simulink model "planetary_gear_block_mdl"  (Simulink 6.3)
settings: Solver=ode45  StartTime=0.0  StopTime=3  RelTol=1e-3
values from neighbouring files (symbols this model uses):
  b_c = kb*J_c    (= 92.8974810391)    [architetture_epicicloidale_statico.m]    (also in architetture_HEV_startstop_1.m = 9.28974810391; architetture_HEV_startstop_2.m = 9.28974810391; architetture_epicicloidale.m = 4.94590955184; architetture_epicicloidale_cont.m = 4.94590955184)
  b_p = kb*J_p    (= 8.12277148259)    [architetture_epicicloidale_statico.m]    (also in architetture_HEV_startstop_1.m = 0.812277148259; architetture_HEV_startstop_2.m = 0.812277148259; CVT_New.m = 0.00430287434624; CVT_New_th.m = 0.00430287434624)
  b_r = kb*J_r    (= 218.026030555)    [architetture_epicicloidale_statico.m]    (also in architetture_HEV_startstop_1.m = 21.8026030555; architetture_HEV_startstop_2.m = 21.8026030555; CVT_New.m = 0.218026030555; CVT_New_th.m = 0.218026030555)
  b_s = kb*J_s    (= 4.94590955184)    [architetture_epicicloidale_statico.m]    (also in architetture_HEV_startstop_1.m = 0.494590955184; architetture_HEV_startstop_2.m = 0.494590955184; CVT_New.m = 0.0104441563023; CVT_New_th.m = 0.0104441563023)
  d_cr = d0    (= 1000)    [architetture_HEV_startstop_1.m]    (also in architetture_HEV_startstop_2.m; architetture_epicicloidale_HEV.m = 10; architetture_HEV_controllo.m; architetture_HEV_startstop.m = 90)
  d_sc = d0    (= 1000)    [architetture_HEV_startstop_1.m]    (also in architetture_HEV_startstop_2.m; architetture_epicicloidale_HEV.m = 10; architetture_HEV_controllo.m; architetture_HEV_startstop.m = 90)
  J_c = Nr_sat*(r_s+r_p)^2*rho_acc*pi*(hs*r_p^2 + hc*r_p^2)    (= 0.928974810391)    [architetture_epicicloidale_statico.m]    (also in architetture_HEV_startstop_1.m; architetture_HEV_startstop_2.m; architetture_epicicloidale.m = 0.0494590955184; architetture_epicicloidale_cont.m = 0.0494590955184)
  J_p = Nr_sat*0.5*pi*rho_acc*(hs*r_p^4 + hc*r_p^4)    (= 0.0812277148259)    [architetture_epicicloidale_statico.m]    (also in architetture_HEV_startstop_1.m; architetture_HEV_startstop_2.m; CVT_New.m = 4.30287434624e-05; CVT_New_th.m = 4.30287434624e-05)
  J_r = 0.5*pi*rho_acc*(hr*r_r^4 + h_ring*(r_re^4-r_r^4))    (= 2.18026030555)    [architetture_epicicloidale_statico.m]    (also in architetture_HEV_startstop_1.m; architetture_HEV_startstop_2.m; CVT_New.m = 0.00218026030555; CVT_New_th.m = 0.00218026030555)
  J_s = 1.3*0.5*pi*rho_acc*hc*r_s^4    (= 0.0494590955184)    [architetture_epicicloidale_statico.m]    (also in architetture_HEV_startstop_1.m; architetture_HEV_startstop_2.m; CVT_New.m = 0.000104441563023; CVT_New_th.m = 0.000104441563023)
  K_cr = K0    (= 10000000)    [architetture_HEV_startstop_1.m]    (also in architetture_HEV_startstop_2.m; architetture_epicicloidale_HEV.m = 10000; architetture_HEV_controllo.m = 100000; architetture_HEV_startstop.m)
  K_sc = K0    (= 10000000)    [architetture_HEV_startstop_1.m]    (also in architetture_HEV_startstop_2.m; architetture_epicicloidale_HEV.m = 10000; architetture_HEV_controllo.m = 100000; architetture_HEV_startstop.m)
  Nr_sat = 4    [architetture_epicicloidale_statico.m]    (also in architetture_HEV_startstop_1.m; architetture_HEV_startstop_2.m; architetture_epicicloidale.m; architetture_epicicloidale_cont.m)
  r_p = xds*Np/(2*pi)    (= 0.0732112738223)    [architetture_epicicloidale_statico.m]    (also in architetture_HEV_startstop_1.m; architetture_HEV_startstop_2.m; CVT_New.m = 0.105042262441; CVT_New_th.m = 0.105042262441)
  r_r = xds*Nr/(2*pi)    (= 0.248281711223)    [architetture_epicicloidale_statico.m]    (also in architetture_HEV_startstop_1.m; architetture_HEV_startstop_2.m; architetture_epicicloidale_HEV.m; architetture_HEV_controllo.m)
  r_s = r_r-2*r_p    (= 0.101859163579)    [architetture_epicicloidale_statico.m]    (also in architetture_HEV_startstop_1.m; architetture_HEV_startstop_2.m; architetture_epicicloidale.m = 0.0732112738223; architetture_epicicloidale_cont.m = 0.0732112738223)
  Tau_c = 0*N*metri    (= 0)    [architetture_epicicloidale_statico.m]    (also in architetture_epicicloidale.m; architetture_epicicloidale_cont.m; architetture_epicicloidale_prova.m; epicicloidale.m)
  Tau_r = 0*N*metri    (= 0)    [architetture_epicicloidale_statico.m]    (also in architetture_epicicloidale.m; architetture_epicicloidale_cont.m; architetture_epicicloidale_prova.m; epicicloidale.m)
  Tau_s = 5*N*metri    (= 5)    [epicicloidale_confronto_statico_elastico.m]    (also in epicicloidale_statico.m = 0)
  Tc = 0.05*ms    (= 5e-05)    [architetture_epicicloidale_statico.m]    (also in architetture_HEV_startstop_1.m; architetture_HEV_startstop_2.m; CVT_New.m; CVT_New_th.m)
  Wc_0 = -0*0.2*rad/secondo    (= 0)    [architetture_epicicloidale_statico.m]    (also in architetture_epicicloidale.m; architetture_epicicloidale_cont.m; architetture_epicicloidale_HEV.m; architetture_epicicloidale_prova.m)
  Wr_0 = WW_0(5),    [CVT_New.m]    (also in CVT_New_th.m; architetture_epicicloidale.m = Sys1.C(3,:)*[Wc_0; Wsc_0]; Confronto_CVT_EMR.m = 0; epicicloidale.m = Sys1.C(3,:)*[Wc_0; Wsc_0])
  Ws_0 = 0*0.1*rad/secondo    (= 0)    [architetture_epicicloidale_statico.m]    (also in epicicloidale_confronto_statico_elastico.m = 0.1; epicicloidale_statico.m = 0.1)
undefined symbols (not defined in the file or in its folder): Tau3, W1, W2

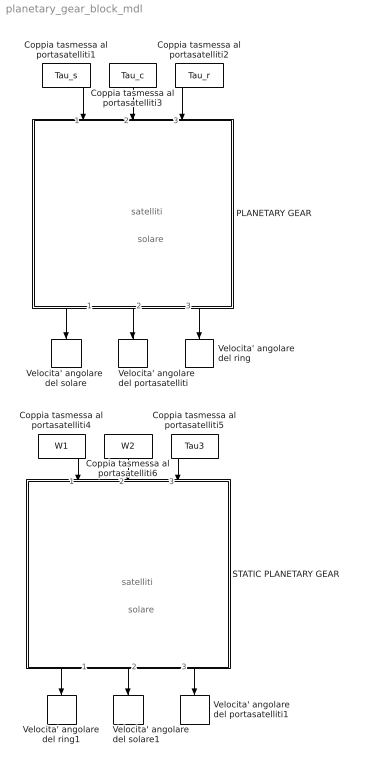
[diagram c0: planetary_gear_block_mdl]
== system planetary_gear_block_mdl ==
  note: solare
  note: satelliti
  note: solare
  note: satelliti
  Coppia tasmessa al portasatelliti1 : Constant  Orientation=down  Value=Tau_s
  Coppia tasmessa al portasatelliti2 : Constant  Orientation=down  Value=Tau_r
  Coppia tasmessa al portasatelliti3 : Constant  Orientation=down  Value=Tau_c
  Coppia tasmessa al portasatelliti4 : Constant  Orientation=down  Value=W1
  Coppia tasmessa al portasatelliti5 : Constant  Orientation=down  Value=Tau3
  Coppia tasmessa al portasatelliti6 : Constant  Orientation=down  Value=W2
  PLANETARY GEAR : Subsystem  Orientation=down  mask(POG Gruppo epicicloidale){Par_solare=[J_s, b_s, r_s], Par_satelliti=[J_p, J_c, b_p, b_c, r_p, Nr_sat], Par_ring=[J_r, b_r, r_r], Tipo_di_Modello=Modello ridotto Ws-Wc, Cond_in_Ws_Wc=[Ws_0,  Wc_0], Cond_in_Wc_Wr=[Wc_0,  Wr_0], Cond_in_Ws_Wr=[Ws_0,  Wr_0], Solare_Satelliti=[K_sc, d_sc], Satelliti_Ring=[K_cr, d_cr], Cond_in=[Ws_0, Wc_0, Wr_0]}
      mask prompts: Par_solare "Parametri Solare: [J_s, b_s, r_s]-->[kg*m^2,N*m*s/rad,m]"; Par_satelliti "Parametri Satelliti: [J_p, J_c, b_p, b_c, r_p, Nr_sat]-->[kg*m^2,N*m*s/rad,m]"; Par_ring "Parametri Ring: [J_r, b_r, r_r]-->[kg*m^2,N*m*s/rad,m,m]"; Tipo_di_Modello "Tipo di modello"; Cond_in_Ws_Wc "Condizioni iniziali: [Ws_0,  Wc_0]-->[rad/s]"; Cond_in_Wc_Wr "Condizioni iniziali: [Wc_0,  Wr_0]-->[rad/s]"; Cond_in_Ws_Wr "Condizioni iniziali: [Ws_0,  Wr_0]-->[rad/s]"; Solare_Satelliti "Solare-Satelliti: [K_sc, d_sc]-->[N/m,N*m*s/rad]"; Satelliti_Ring "Satelliti-Ring: [K_cr, d_cr]-->[N/m,N*m*s/rad]"; Cond_in "Condizioni iniziali: [Ws_0,  Wc_0, Wr_0]-->[rad/s]"
      mask help: Gruppo epicicloidale: [J_s, J_p, J_c, J_r]= Inerzie di: solare, satelliti, porta-satelliti, ring; [b_s, b_p, b_c, b_r]= Attriti di: solare, satelliti, porta-satelliti, ring; [r_s, r_p, r_r]= Raggi di: solare, satelliti, ring; [Nr_sat]= Numero Satelliti; [K_sc, K_cr]= Elasticita' tra solare-satelliti e tra satelliti-ring; [d_sc, d_cr]= Elementi della matrice D; [Ws_0, Wc_0, Wr_0]=Velocita' iniziali di solare, porta-satelliti, ring;
      mask init:
      | J_s=double(Par_solare(1));          
      | b_s=double(Par_solare(2));            
      | r_s=double(Par_solare(3));           
      | %
      | J_p=double(Par_satelliti(1));            
      | J_c=double(Par_satelliti(2));            
      | b_p=double(Par_satelliti(3));            
      | b_c=double(Par_satelliti(4));            
      | r_p=double(Par_satelliti(5));            
      | Nr_sat=double(Par_satelliti(6));           
      | %
      | J_r=double(Par_ring(1));             
      | b_r=double(Par_ring(2));            
      | r_r=double(Par_ring(3));                  
      | %
      | %%%%%%%%%%%%%%%%%%%%%%%%%%%%%%%%%%%%%%%%%%%%%%%%%%%%%%%%%%%%%%%%%%%%%%%%%%%
      | %   Modello esteso e modelli ridotti
      | %%%%%%%%%%%%%%%%%%%%%%%%%%%%%%%%%%%%%%%%%%%%%%%%%%%%%%%%%%%%%%%%%%%%%%%%%%%
      | if Tipo_di_Modello=='Modello esteso       '
      |     %
      |     K_sc=double(Solare_Satelliti(1));
      |     d_sc=double(Solare_Satelliti(2));
      |     if(K_sc==0)
      |         K_sc=inf;
      |     end
      |     %
      |     K_cr=double(Satelliti_Ring(1));
      |     d_cr=double(Satelliti_Ring(2));
      |     if(K_cr==0)
      |         K_cr=inf;
      |     end
      |     %
      |     %
      |     L=[ J_s,    0,      0,      0,      0,      0;
      |         0, 1/K_sc,      0,      0,      0,      0;
      |         0,      0,    J_p,      0,      0,      0;
      |         0,      0,      0,    J_c,      0,      0;
      |         0,      0,      0,      0, 1/K_cr,      0;
      |         0,      0,      0,      0,      0,    J_r];
      |     %
      |     A=- [-b_s-r_s^2*d_sc,                       -r_s,              -r_s*d_sc*r_p,                 r_s^2*d_sc,                          0,                          0;
      |                         r_s,                          0,                        r_p,                       -r_s,                          0,                          0;
      |               -r_s*d_sc*r_p,                       -r_p, -b_p-d_sc*r_p^2-d_cr*r_p^2,  r_s*d_sc*r_p-d_cr*r_p*r_r,                       -r_p,               d_cr*r_p*r_r;
      |                  r_s^2*d_sc,                        r_s,  r_s*d_sc*r_p-d_cr*r_p*r_r, -b_c-r_s^2*d_sc-d_cr*r_r^2,                       -r_r,                 d_cr*r_r^2;
      |                           0,                          0,                        r_p,                        r_r,                          0,                       -r_r;
      |                           0,                          0,               d_cr*r_p*r_r,                 d_cr*r_r^2,                        r_r,            -b_r-d_cr*r_r^2];
      | %                         
      |     B=[ 1, 0, 0;
      |         0, 0, 0;
      |         0, 0, 0;
      |         0, 1, 0;
      |         0, 0, 0;
      |         0, 0, 1];
      |     %
      |     C=[ 1, 0, 0, 0, 0, 0;
      |         0, 0, 0, 1, 0, 0;
      |         0, 0, 0, 0, 0, 1];
      |     %
      |     Ws_0=double(Cond_in(1));
      |     Wc_0=double(Cond_in(2));
      |     Wr_0=double(Cond_in(3));
      |     Wp_0=r_s*(Wc_0-Ws_0)/r_p;
      |     Wpc_0=[Wp_0 Wc_0];
      |     %
      |     We_0=[Ws_0 0 Wpc_0 0 Wr_0 ];
      |     %
      | elseif Tipo_di_Modello=='Modello ridotto Ws-Wc'
      |     L = [(J_s*r_p^2*r_r^2+r_s^2*J_p*r_r^2+r_s^2*J_r*r_p^2)/r_p^2/r_r^2,                                      -r_s*(r_s*J_p*r_r^2+J_r*r_p^2*r_s+J_r*r_p^2*r_r)/r_p^2/r_r^2;
      |            -r_s*(r_s*J_p*r_r^2+J_r*r_p^2*r_s+J_r*r_p^2*r_r)/r_p^2/r_r^2, (J_c*r_p^2*r_r^2+r_s^2*J_p*r_r^2+r_s^2*J_r*r_p^2+2*J_r*r_p^2*r_s*r_r+J_r*r_p^2*r_r^2)/r_p^2/r_r^2];
      |     %
      |     A=-[ -(b_s*r_p^2*r_r^2+r_s^2*b_p*r_r^2+r_s^2*b_r*r_p^2)/r_p^2/r_r^2,                                        r_s*(r_s*b_p*r_r^2+b_r*r_p^2*r_s+b_r*r_p^2*r_r)/r_p^2/r_r^2;
      |         r_s*(r_s*b_p*r_r^2+b_r*r_p^2*r_s+b_r*r_p^2*r_r)/r_p^2/r_r^2, -(b_c*r_p^2*r_r^2+r_s^2*b_p*r_r^2+r_s^2*b_r*r_p^2+2*b_r*r_p^2*r_s*r_r+b_r*r_p^2*r_r^2)/r_p^2/r_r^2];
      |     %
      |     B= [  1,             0,    -1/r_r*r_s;
      |            0,             1, (r_s+r_r)/r_r];
      |     %
      |     C= [            1,               0;
      |                     0,               1;
      |            -1/r_r*r_s, (r_s+r_r)/r_r];
      |     %
      |     Ws_0=double(Cond_in_Ws_Wc(1));
      |     Wc_0=double(Cond_in_Ws_Wc(2));
      |     We_0=[Ws_0 Wc_0];
      |     %
      | elseif Tipo_di_Modello=='Modello ridotto Wc-Wr'
      |     L= [ (J_c*r_s^2*r_p^2+J_s*r_p^2*r_s^2+2*J_s*r_p^2*r_s*r_r+J_s*r_p^2*r_r^2+r_r^2*J_p*r_s^2)/r_s^2/r_p^2,                                      -r_r*(J_s*r_p^2*r_s+J_s*r_p^2*r_r+r_r*J_p*r_s^2)/r_s^2/r_p^2;
      |           -r_r*(J_s*r_p^2*r_s+J_s*r_p^2*r_r+r_r*J_p*r_s^2)/r_s^2/r_p^2,                                     (J_r*r_s^2*r_p^2+J_s*r_p^2*r_r^2+r_r^2*J_p*r_s^2)/r_s^2/r_p^2];
      | 
      |     A=-[  -(b_c*r_s^2*r_p^2+b_s*r_p^2*r_s^2+2*b_s*r_p^2*r_s*r_r+b_s*r_p^2*r_r^2+r_r^2*b_p*r_s^2)/r_s^2/r_p^2,                                        r_r*(b_s*r_p^2*r_s+b_s*r_p^2*r_r+r_r*b_p*r_s^2)/r_s^2/r_p^2;
      |          r_r*(b_s*r_p^2*r_s+b_s*r_p^2*r_r+r_r*b_p*r_s^2)/r_s^2/r_p^2,                                     -(b_r*r_s^2*r_p^2+b_s*r_p^2*r_r^2+r_r^2*b_p*r_s^2)/r_s^2/r_p^2];
      | 
      |     B= [ (r_s+r_r)/r_s,    1,   0;
      |             -1/r_s*r_r,    0,   1];
      | 
      |     C= [ (r_s+r_r)/r_s,    -1/r_s*r_r;
      |                       1,            0;
      |                       0,            1];
      |     %
      |     Wc_0=double(Cond_in_Wc_Wr(1));
      |     Wr_0=double(Cond_in_Wc_Wr(2));
      |     We_0=[Wc_0 Wr_0];
      |     %
      | elseif Tipo_di_Modello=='Modello ridotto Ws-Wr'
      |     L= [ (J_c*r_s^2*r_p^2+J_s*r_p^2*r_s^2+2*J_s*r_p^2*r_s*r_r+J_s*r_p^2*r_r^2+r_r^2*J_p*r_s^2)/r_p^2/(r_s+r_r)^2,                                                      -r_s*r_r*(r_r*J_p*r_s-J_c*r_p^2)/r_p^2/(r_s+r_r)^2;
      |           -r_s*r_r*(r_r*J_p*r_s-J_c*r_p^2)/r_p^2/(r_s+r_r)^2, (J_r*r_s^2*r_p^2+2*J_r*r_p^2*r_s*r_r+J_r*r_p^2*r_r^2+r_r^2*J_p*r_s^2+r_r^2*J_c*r_p^2)/r_p^2/(r_s+r_r)^2];
      | 
      |     A=-[-(b_c*r_s^2*r_p^2+b_s*r_p^2*r_s^2+2*b_s*r_p^2*r_s*r_r+b_s*r_p^2*r_r^2+r_r^2*b_p*r_s^2)/r_p^2/(r_s+r_r)^2,                                                      -r_s*r_r*(-r_s*r_r*b_p+r_p^2*b_c)/r_p^2/(r_s+r_r)^2;
      |                                                               -r_s*r_r*(-r_s*r_r*b_p+r_p^2*b_c)/r_p^2/(r_s+r_r)^2, -(b_r*r_p^2*r_s^2+2*b_r*r_p^2*r_s*r_r+b_r*r_p^2*r_r^2+r_r^2*b_p*r_s^2+r_r^2*r_p^2*b_c)/r_p^2/(r_s+r_r)^2];
      | 
      |     B=[   1,  1/(r_s+r_r)*r_s, 0;
      |           0, 1/(r_s+r_r)*r_r, 1];
      | 
      |     C=[                 1,                  0;
      |          1/(r_s+r_r)*r_s, 1/(r_s+r_r)*r_r;
      |                         0,                  1];
      |     Ws_0=double(Cond_in_Ws_Wr(1));
      |     Wr_0=double(Cond_in_Ws_Wr(2));
      |     We_0=[Ws_0 Wr_0];
      | end
  STATIC PLANETARY GEAR : Subsystem  Orientation=down  mask(POG Gruppo epicicloidale){Raggi_sun_ring=[r_s, r_r], Tipo_di_Modello=Modello ridotto Ws-Wc, Cond_in_Ws_Wc=[Ws_0,  Wc_0], Cond_in_Wc_Wr=[Wc_0,  Wr_0], Cond_in_Ws_Wr=[Ws_0,  Wr_0], Cond_in=[Ws_0, Wc_0, Wr_0]}
      mask prompts: Raggi_sun_ring "Raggi Sun, Ring: [r_s, r_r]-->[m,m]"; Tipo_di_Modello "Tipo di modello"; Cond_in_Ws_Wc "Condizioni iniziali: [Ws_0,  Wc_0]-->[rad/s]"; Cond_in_Wc_Wr "Condizioni iniziali: [Wc_0,  Wr_0]-->[rad/s]"; Cond_in_Ws_Wr "Condizioni iniziali: [Ws_0,  Wr_0]-->[rad/s]"; Cond_in "Condizioni iniziali: [Ws_0,  Wc_0, Wr_0]-->[rad/s]"
      mask help: Gruppo epicicloidale: [r_s, r_r]= Raggi di: sun e ring; [Ws_0, Wc_0, Wr_0]=Velocita' iniziali di sun, carrieri, ring;
      mask init:
      | r_s=Raggi_sun_ring(1);
      | r_r=Raggi_sun_ring(2);
      | 
      | %
      | %%%%%%%%%%%%%%%%%%%%%%%%%%%%%%%%%%%%%%%%%%%%%%%%%%%%%%%%%%%%%%%%%%%%%%%%%%%
      | %   Modello statico tutti i casi
      | %%%%%%%%%%%%%%%%%%%%%%%%%%%%%%%%%%%%%%%%%%%%%%%%%%%%%%%%%%%%%%%%%%%%%%%%%%%
      | if Tipo_di_Modello=='Modello ridotto Ws-Wc'
      |       %
      |     B= [ -1/r_r*r_s,  (r_s+r_r)/r_r];
      |     %
      |     Ws_0=double(Cond_in_Ws_Wc(1));
      |     Wc_0=double(Cond_in_Ws_Wc(2));
      |     We_0=[Ws_0 Wc_0];
      |     %
      | elseif Tipo_di_Modello=='Modello ridotto Wc-Wr'
      |     B= [ (r_s+r_r)/r_s,  -1/r_s*r_r];
      |    %
      |     Wc_0=double(Cond_in_Wc_Wr(1));
      |     Wr_0=double(Cond_in_Wc_Wr(2));
      |     We_0=[Wc_0 Wr_0];
      |     %
      | elseif Tipo_di_Modello=='Modello ridotto Ws-Wr'
      |  
      |     B=[1/(r_s+r_r)*r_s, 1/(r_s+r_r)*r_r];
      |    %
      |     Ws_0=double(Cond_in_Ws_Wr(1));
      |     Wr_0=double(Cond_in_Ws_Wr(2));
      |     We_0=[Ws_0 Wr_0];
      | end
  Velocita' angolare del ring : ToWorkspace  VariableName=Wr  SampleTime=Tc  SaveFormat=Array
  Velocita' angolare del ring1 : ToWorkspace  VariableName=W3  SampleTime=Tc  SaveFormat=Array
  Velocita' angolare  del portasatelliti : ToWorkspace  VariableName=Wc  SampleTime=Tc  SaveFormat=Array
  Velocita' angolare  del portasatelliti1 : ToWorkspace  VariableName=Tau2  SampleTime=Tc  SaveFormat=Array
  Velocita' angolare  del solare : ToWorkspace  VariableName=Ws  SampleTime=Tc  SaveFormat=Array
  Velocita' angolare  del solare1 : ToWorkspace  VariableName=Tau1  SampleTime=Tc  SaveFormat=Array
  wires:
  PLANETARY GEAR/3(Wr) -> Velocita' angolare del ring/1
  PLANETARY GEAR/2(Wc) -> Velocita' angolare  del portasatelliti/1
  PLANETARY GEAR/1(Ws) -> Velocita' angolare  del solare/1
  Coppia tasmessa al portasatelliti1/1 -> PLANETARY GEAR/1(Ts)
  Coppia tasmessa al portasatelliti2/1 -> PLANETARY GEAR/3(Tr)
  Coppia tasmessa al portasatelliti3/1 -> PLANETARY GEAR/2(Tc)
  STATIC PLANETARY GEAR/1(Tau1) -> Velocita' angolare del ring1/1
  STATIC PLANETARY GEAR/3(W3) -> Velocita' angolare  del portasatelliti1/1
  STATIC PLANETARY GEAR/2(Tau2) -> Velocita' angolare  del solare1/1
  Coppia tasmessa al portasatelliti4/1 -> STATIC PLANETARY GEAR/1(W1)
  Coppia tasmessa al portasatelliti5/1 -> STATIC PLANETARY GEAR/3(Tau3)
  Coppia tasmessa al portasatelliti6/1 -> STATIC PLANETARY GEAR/2(W2)

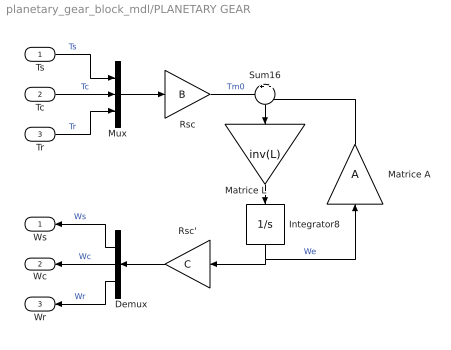
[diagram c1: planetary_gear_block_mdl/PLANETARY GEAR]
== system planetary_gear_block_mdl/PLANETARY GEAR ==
  Ts : Inport
  Tc : Inport  Port=2
  Tr : Inport  Port=3
  Demux : Demux  Orientation=left  Outputs=3
  Integrator8 : Integrator  Orientation=down  InitialCondition=We_0  LowerSaturationLimit=0
  Matrice A : Gain  Orientation=up  Gain=A  Multiplication=Matrix(K*u)
  Matrice L : Gain  Orientation=down  Gain=inv(L)  Multiplication=Matrix(K*u)
  Mux : Mux  Inputs=3
  Rsc : Gain  Gain=B  Multiplication=Matrix(K*u)
  Rsc' : Gain  Orientation=left  Gain=C  Multiplication=Matrix(K*u)
  Sum16 : Sum  Orientation=down  Inputs=+|-
  Ws : Outport  Orientation=left
  Wc : Outport  Orientation=left  Port=2
  Wr : Outport  Orientation=left  Port=3
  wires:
  Rsc/1 -> Sum16/1  "Tm0"
  Sum16/1 -> Matrice L/1
  Matrice L/1 -> Integrator8/1
  Integrator8/1 -> Matrice A/1, Rsc'/1  "We"
  Matrice A/1 -> Sum16/2
  Ts/1 -> Mux/1  "Ts"
  Tc/1 -> Mux/2  "Tc"
  Tr/1 -> Mux/3  "Tr"
  Mux/1 -> Rsc/1
  Rsc'/1 -> Demux/1
  Demux/1 -> Ws/1  "Ws"
  Demux/2 -> Wc/1  "Wc"
  Demux/3 -> Wr/1  "Wr"

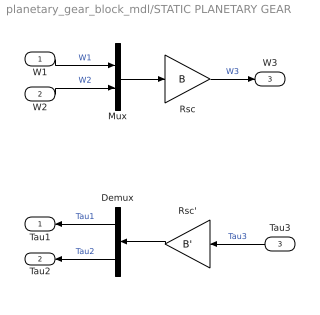
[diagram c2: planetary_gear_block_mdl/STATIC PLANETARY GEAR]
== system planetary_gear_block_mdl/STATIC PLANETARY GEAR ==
  W1 : Inport
  W2 : Inport  Port=2
  Tau3 : Inport  Orientation=left  Port=3
  Demux : Demux  Orientation=left  Outputs=2
  Mux : Mux  Inputs=2
  Rsc : Gain  Gain=B  Multiplication=Matrix(K*u)
  Rsc' : Gain  Orientation=left  Gain=B'  Multiplication=Matrix(K*u)
  Tau1 : Outport  Orientation=left
  Tau2 : Outport  Orientation=left  Port=2
  W3 : Outport  Port=3
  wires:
  Demux/2 -> Tau2/1  "Tau2"
  Demux/1 -> Tau1/1  "Tau1"
  Rsc'/1 -> Demux/1
  Mux/1 -> Rsc/1
  W2/1 -> Mux/2  "W2"
  W1/1 -> Mux/1  "W1"
  Rsc/1 -> W3/1  "W3"
  Tau3/1 -> Rsc'/1  "Tau3"
